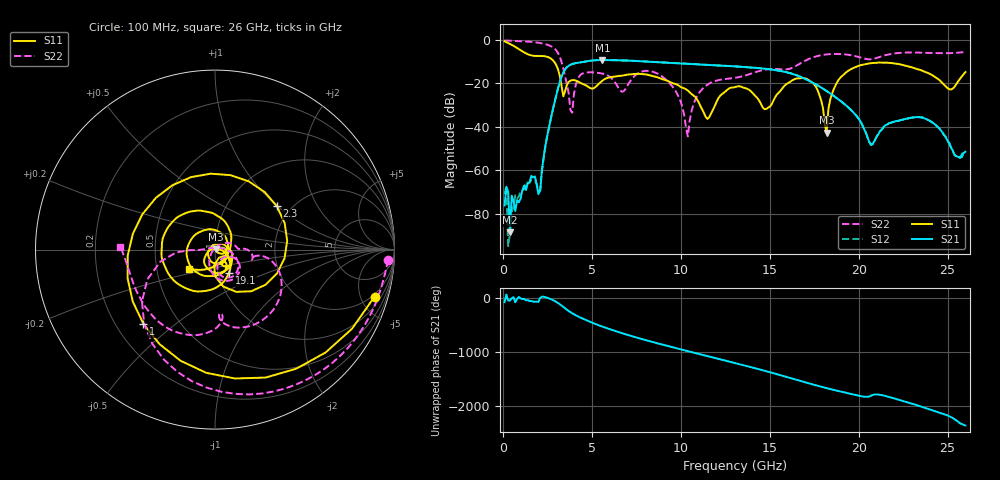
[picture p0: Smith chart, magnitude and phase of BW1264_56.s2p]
!Keysight Technologies,N5245B,MY57181159,A.13.60.06
!Date: Friday, December 18, 2020 23:54:59
!Correction: S11(Full 2 Port(1,2))
!S21(Full 2 Port(1,2))
!S12(Full 2 Port(1,2))
!S22(Full 2 Port(1,2))
!S2P File: Measurements: S11, S21, S12, S22:
# Hz S  dB  R 50
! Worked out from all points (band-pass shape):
!   260 points, 100 MHz to 26 GHz, reference 50 ohm
!   highest |S21| = -9.32 dB at 5.6 GHz (marker M1); lowest = -88.5 dB at 400 MHz (marker M2)
!   |S21| within 3 dB of the highest: 3.644 GHz to 13.23 GHz (9.588 GHz wide, 114 % of centre)
!   lowest |S11| = -42.7 dB at 18.2 GHz (marker M3), VSWR 1.01, Z = 50.7 + j0.167 ohm
!   |S11| at or under -10 dB: 2.875 GHz to end of sweep
!   |S22| runs from -44.4 to -0.3 dB; largest |S21 - S12| = 0.00059
!   S11 on the Smith chart (normalised r, x): 100 MHz: 1.74, -6.48; 1 GHz: 0.31, -0.39; 2.3 GHz: 1.69, +0.99; 19.1 GHz: 1.13, -0.30; 26 GHz: 0.73, -0.16
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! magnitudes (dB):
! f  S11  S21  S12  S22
! 100 MHz  -0.7  -76.2  -71.0  -0.3
! 200 MHz  -1.1  -67.6  -67.2  -0.4
! 400 MHz  -1.9  -88.5  -89.0  -0.4
! 1 GHz  -4.8  -73.0  -69.7  -0.6
! 2 GHz  -7.5  -71.0  -69.6  -1.4
! 2.3 GHz  -7.5  -53.5  -54.2  -1.8
! 3.2 GHz  -16.5  -19.5  -19.5  -7.7
! 3.9 GHz  -18.6  -11.2  -11.2  -33.5
! 4.5 GHz  -20.3  -10.2  -10.2  -15.4
! 5.6 GHz  -18.8  -9.3  -9.3  -15.5
! 8.8 GHz  -17.6  -10.4  -10.4  -16.1
! 10.4 GHz  -23.4  -11.0  -11.0  -44.4
! 11.5 GHz  -36.4  -11.5  -11.5  -20.7
! 13.1 GHz  -21.6  -12.3  -12.3  -17.4
! 14.7 GHz  -31.9  -13.3  -13.3  -13.8
! 17.4 GHz  -19.8  -19.6  -19.6  -8.2
! 18.2 GHz  -42.7  -23.5  -23.6  -6.7
! 18.4 GHz  -27.6  -24.7  -24.7  -6.6
! 19.1 GHz  -16.4  -28.9  -28.9  -6.6
! 20.7 GHz  -10.7  -48.3  -48.5  -8.9
! 21.7 GHz  -10.6  -38.4  -38.4  -6.7
! 26 GHz  -14.8  -51.5  -51.4  -5.6
